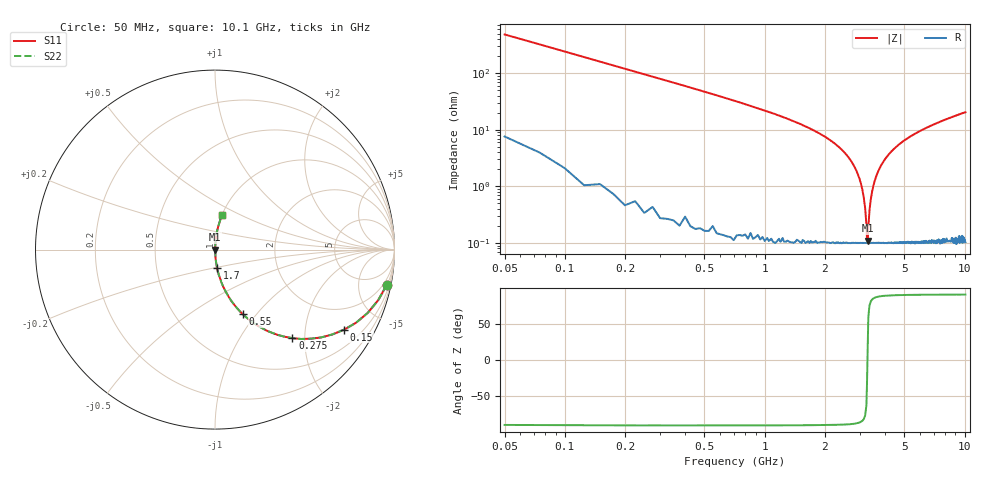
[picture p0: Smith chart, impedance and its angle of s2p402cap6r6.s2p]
! AVX Thin Film Operation		Date: April 2003
! Description: Accu-P® Series, Thin Film, SMD, RF Capacitor
! Part Number: 0402ZK6R6BBW
! 50 MHz  -  10.05 GHz
! Serial Measurements
# hz S db R 50
!	S11		S21		S12		S22
!	dB	Phase	dB	Phase	dB	Phase	dB	Phase
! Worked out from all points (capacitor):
!   400 points, 50 MHz to 10.1 GHz, reference 50 ohm
!   read as one part in series: C = 6.6 pF near 100 MHz
!   lowest |Z| = 110 mohm at 3.28 GHz (marker M1)
!   series resonance near 3.268 GHz, so ESL is about 360 pH
!   S11 on the Smith chart (normalised r, x): 50 MHz: 1.15, -9.62; 150 MHz: 1.02, -3.21; 275 MHz: 1.01, -1.74; 550 MHz: 1.00, -0.85; 1.7 GHz: 1.00, -0.21; 10.1 GHz: 1.00, +0.41
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5e7  -0.21 -11.7  -13.90 77.4  -13.90 77.4  -0.21 -11.7
1.5e8  -1.45 -31.8  -5.55 57.8  -5.55 57.8  -1.45 -31.8
2.75e8  -3.67 -48.8  -2.47 40.9  -2.47 40.9  -3.67 -48.8
5.5e8  -8.15 -66.7  -0.74 23.0  -0.74 23.0  -8.15 -66.7
1.7e9  -19.80 -83.5  -0.06 5.9  -0.06 5.9  -19.80 -83.5
1.73e9  -20.00 -83.7  -0.05 5.8  -0.05 5.8  -20.00 -83.7
2.43e9  -27.00 -86.2  -0.02 2.5  -0.02 2.5  -27.00 -86.2
2.88e9  -34.50 -85.9  -0.01 1.1  -0.01 1.1  -34.50 -85.9
3.13e9  -43.70 -80.9  -0.01 0.4  -0.01 0.4  -43.70 -80.9
3.18e9  -47.40 -76.2  -0.01 0.2  -0.01 0.2  -47.40 -76.2
3.23e9  -53.60 -61.2  -0.01 0.1  -0.01 0.1  -53.60 -61.2
3.25e9  -58.30 -34.4  -0.01 0.0  -0.01 0.0  -58.30 -34.4
3.28e9  -59.20 24.1  -0.01 -0.0  -0.01 -0.0  -59.20 24.1
3.3e9  -54.60 57.4  -0.01 -0.1  -0.01 -0.1  -54.60 57.4
3.35e9  -48.10 75.0  -0.01 -0.2  -0.01 -0.2  -48.10 75.0
3.4e9  -44.40 80.2  -0.01 -0.3  -0.01 -0.3  -44.40 80.2
3.55e9  -38.10 84.7  -0.01 -0.7  -0.01 -0.7  -38.10 84.7
3.85e9  -32.20 86.3  -0.01 -1.4  -0.01 -1.4  -32.20 86.3
5.08e9  -23.50 85.3  -0.03 -3.9  -0.03 -3.9  -23.50 85.3
6.75e9  -18.70 82.8  -0.07 -6.7  -0.07 -6.7  -18.70 82.8
8.43e9  -15.90 80.4  -0.12 -9.2  -0.12 -9.2  -15.90 80.4
1.01e10  -14.00 78.2  -0.18 -11.5  -0.18 -11.5  -14.00 78.2
